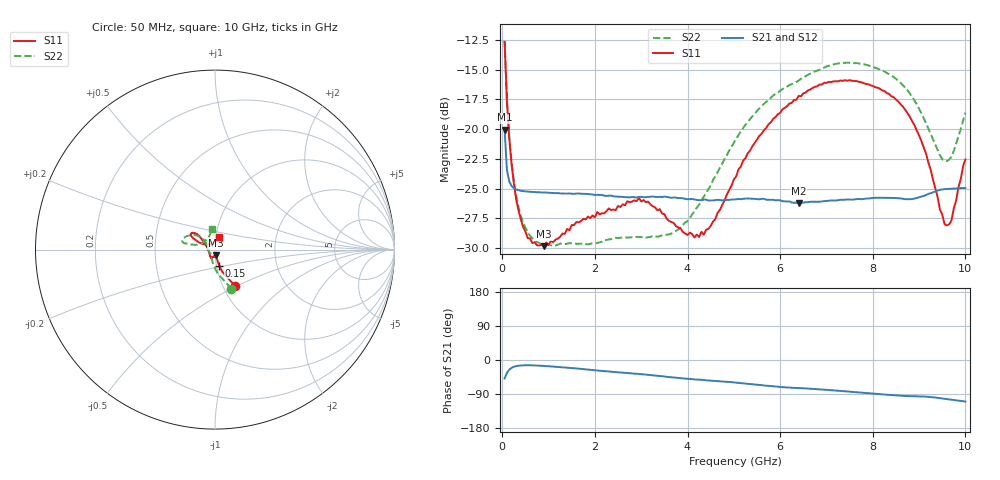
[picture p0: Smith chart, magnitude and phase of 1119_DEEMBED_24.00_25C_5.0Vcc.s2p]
!Hittite Microwave Corp.
!Digital Attenuator/PhaseShifter Rev 1.4.0
!Filename: C:\DATA\DATA\1119_DEEMBED_24.00_25C_5.0Vcc.s2p
!VNA ID: Agilent Technologies,N5224A,MY51441122,A.10.45.03
!Device type:
!2 Port Calibration.
!Temp(C): 25
!Lot Number:
!Serial Number:
!Operator:
!Misc:
!Attenuator:  24.000
# GHZ S DB R 50.0
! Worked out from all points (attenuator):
!   200 points, 50 MHz to 10 GHz, reference 50 ohm
!   highest |S21| = -20.05 dB at 50 MHz (marker M1); lowest = -26.2 dB at 6.4 GHz (marker M2)
!   lowest |S11| = -29.9 dB at 900 MHz (marker M3), VSWR 1.07, Z = 50.2 - j3.22 ohm
!   |S11| at or under -10 dB: start of sweep to end of sweep
!   |S22| runs from -29.8 to -12.6 dB; largest |S21 - S12| = 0.00019
!   S11 on the Smith chart (normalised r, x): 50 MHz: 1.14, -0.49; 150 MHz: 1.03, -0.18; 10 GHz: 1.04, +0.15
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0.05  -12.69 -61.1  -20.05 -48.6  -20.06 -48.7  -12.55 -67.3
0.1  -17.65 -71.7  -23.45 -34.0  -23.45 -34.0  -17.51 -83.8
0.15  -20.73 -75.4  -24.40 -25.4  -24.41 -25.4  -20.64 -93.3
0.3  -25.92 -77.7  -25.08 -16.2  -25.08 -16.2  -25.59 -110.4
0.45  -28.24 -77.5  -25.22 -14.1  -25.22 -14.0  -27.87 -121.2
0.9  -29.85 -84.2  -25.34 -15.6  -25.34 -15.7  -29.76 -135.6
1.75  -27.55 -102.8  -25.45 -24.2  -25.46 -24.2  -29.65 -140.5
2.95  -25.79 -114.4  -25.71 -36.8  -25.71 -36.9  -29.09 -159.8
3.4  -26.74 -126.4  -25.70 -42.2  -25.71 -42.2  -29.01 -173.3
3.8  -28.28 -141.2  -25.80 -47.3  -25.80 -47.4  -28.44 170.8
4.25  -29.08 -167.5  -25.98 -52.0  -25.99 -52.1  -26.37 152.6
4.6  -27.56 168.1  -25.98 -55.0  -26.00 -55.1  -23.96 143.1
5.05  -23.99 149.4  -25.91 -59.6  -25.92 -59.7  -20.83 138.9
5.55  -20.58 141.4  -25.91 -65.7  -25.93 -65.7  -18.26 141.3
6.4  -17.21 139.9  -26.22 -74.1  -26.24 -74.1  -15.92 150.0
6.7  -16.55 141.8  -26.11 -76.3  -26.12 -76.3  -15.23 154.0
7.5  -15.89 147.8  -25.93 -83.6  -25.94 -83.7  -14.43 163.6
8.35  -17.04 151.9  -25.79 -92.0  -25.80 -92.0  -15.37 168.0
8.999999  -20.54 155.8  -25.74 -95.9  -25.76 -95.9  -18.30 167.3
9.55  -27.99 124.8  -25.05 -102.4  -25.06 -102.4  -22.68 138.1
9.7  -27.68 97.5  -25.02 -104.7  -25.03 -104.7  -22.31 119.9
10  -22.55 71.8  -24.97 -109.6  -24.98 -109.6  -18.62 98.5
